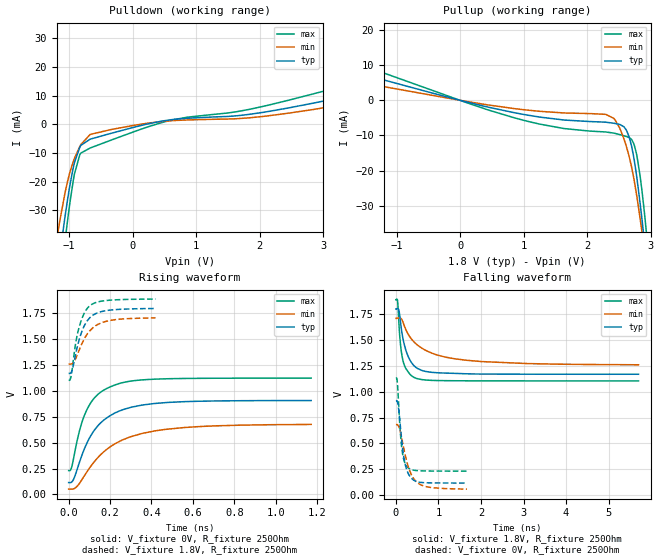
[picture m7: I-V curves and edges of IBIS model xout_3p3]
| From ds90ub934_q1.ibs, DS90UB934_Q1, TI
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|   xout_3p3 Model
[Model]   xout_3p3
Model_type   Output
Polarity   Inverting
Vmeas = 0.9
Vref = 0
Cref = 2pF
Rref = 450
|   typ   min   max
|   (nom PVT)   (fast PVT)   (slow PVT)
C_comp   3.237e-13   3.062e-13   3.274e-13
| Where nom  PVT is Nominal Process, 1.8V, 27C
|   Fast PVT is Strong Process,  1.89V, -40C
|   Slow PVT is Weak Process,   1.71V, 125C
[Voltage Range]   1.8   1.71   1.89
|Junction Temperature
[Temperature Range]   27   125   -40
[Pullup Reference]   1.8   1.71   1.89
[Pulldown Reference]   0   0   0
[Power Clamp Reference]   1.8   1.71   1.89
[GND Clamp Reference]   0   0   0
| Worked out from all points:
|   slope of the pulldown table from 0 to 0.27 V, typ, clamps not added: 188 ohm
|   slope of the pullup table from 0 to 0.27 V, typ, clamps not added: 225 ohm
|   falling waveform, V_fixture 1.8V, R_fixture 250Ohm: 20-80 % time 238ps typ, 803ps min, 133ps max; typ from 1.8 V to 1.17 V
|   rising waveform, V_fixture 0V, R_fixture 250Ohm: 20-80 % time 145ps typ, 217ps min, 101ps max; typ from 0.114 V to 0.907 V
|   rising waveform, V_fixture 1.8V, R_fixture 250Ohm: 20-80 % time 60.1ps typ, 79.4ps min, 50.6ps max; typ from 1.17 V to 1.8 V
|   falling waveform, V_fixture 0V, R_fixture 250Ohm: 20-80 % time 147ps typ, 251ps min, 97.3ps max; typ from 0.91 V to 0.116 V
[Pulldown]
|   Voltage   I(typ)   I(min)   I(max)
-3.3V     -456.4mA   -384.1mA   -520.8mA
-1.191V   -52.42mA   -39.27mA   -64.54mA
-1.063V   -31.71mA   -23.58mA   -40.14mA
-1.024V   -25.97mA   -19.69mA   -33.2mA
-938.4mV  -15.27mA   -13.06mA   -19.82mA
-826.8mV  -7.669mA   -7.408mA   -10.31mA
-670mV    -5.126mA   -3.48mA    -8.212mA
-329.7mV  -3.027mA   -1.717mA   -5.365mA
600.6mV   1.639mA    1.305mA    1.469mA
2.834V    7.407mA    5.197mA    10.63mA
4.26V     14.33mA    11.36mA    19.17mA
6.6V      27.27mA    13.11mA    34.11mA
[Pullup]
|   Voltage   I(typ)   I(min)   I(max)
-3.3V     15.02mA    10.69mA    20.67mA
856.2mV   -3.531mA   -2.361mA   -4.989mA
2.294V    -6.227mA   -3.997mA   -9.007mA
2.44V     -6.587mA   -5.567mA   -9.417mA
2.579V    -7.519mA   -10.94mA   -10.09mA
2.663V    -10.48mA   -16.05mA   -10.61mA
2.733V    -16.04mA   -21.97mA   -12.26mA
2.786V    -22.35mA   -27.65mA   -15.97mA
2.865V    -34.06mA   -37.61mA   -25.95mA
2.906V    -40.77mA   -43.25mA   -32.67mA
2.973V    -52.11mA   -52.77mA   -44.82mA
6.6V      -759.2mA   -658.7mA   -843.5mA
[Ramp]
R_load = 250
|   typ   min   max
dV/dt_r   0.477545/1.46647e-10   0.378028/2.21303e-10  0.537961/1.01561e-10
dV/dt_f   0.377772/2.3846e-10   0.26956/8.15686e-10   0.471638/1.33752e-10
[Falling Waveform]
V_fixture = 1.8V
V_fixture_min = 1.71V
V_fixture_max = 1.89V
R_fixture = 250Ohm
|   Time   V(typ)   V(min)   V(max)
0s        1.8V       1.71V      1.89V
40.63ps   1.806V     1.714V     1.871V
67.86ps   1.793V     1.714V     1.676V
102.7ps   1.689V     1.712V     1.475V
177.7ps   1.49V      1.661V     1.282V
303.3ps   1.327V     1.547V     1.184V
485.1ps   1.231V     1.46V      1.129V
969.9ps   1.185V     1.356V     1.109V
1.671ns   1.174V     1.305V     1.106V
5.704ns   1.17V      1.262V     1.105V
[Rising Waveform]
V_fixture = 0V
V_fixture_min = 0V
V_fixture_max = 0V
R_fixture = 250Ohm
|   Time   V(typ)   V(min)   V(max)
0s        114.4mV    51.01mV    229.9mV
11.63ps   115.4mV    50.33mV    245.5mV
25.05ps   151.2mV    54.71mV    360.7mV
58.81ps   349.1mV    126.1mV    661.8mV
90.21ps   504.1mV    223.9mV    826.9mV
144.9ps   671.1mV    363.6mV    972.7mV
223ps     786.3mV    488mV      1.057V
354.8ps   863.1mV    589.1mV    1.106V
485.1ps   889.2mV    631.8mV    1.118V
1.171ns   907.1mV    676mV      1.124V
[Rising Waveform]
V_fixture = 1.8V
V_fixture_min = 1.71V
V_fixture_max = 1.89V
R_fixture = 250Ohm
|   Time   V(typ)   V(min)   V(max)
0s        1.169V     1.26V      1.103V
11.63ps   1.177V     1.26V      1.141V
20ps      1.224V     1.268V     1.257V
34.22ps   1.359V     1.313V     1.464V
51.99ps   1.503V     1.4V       1.626V
74.92ps   1.627V     1.5V       1.75V
95.94ps   1.692V     1.566V     1.811V
138.8ps   1.754V     1.64V      1.859V
194.7ps   1.78V      1.679V     1.876V
419.7ps   1.797V     1.706V     1.888V
[Falling Waveform]
V_fixture = 0V
V_fixture_min = 0V
V_fixture_max = 0V
R_fixture = 250Ohm
|   Time   V(typ)   V(min)   V(max)
0s        910.3mV    681.1mV    1.127V
20ps      914.2mV    683.4mV    1.128V
34.22ps   903.5mV    681mV      1.083V
95.94ps   700.4mV    624.5mV    645.5mV
138.8ps   518.4mV    545.2mV    447.4mV
199.7ps   332.6mV    421.2mV    322.5mV
256.5ps   240.5mV    320.2mV    276.9mV
419.7ps   142.7mV    156.2mV    240.1mV
604.7ps   121.1mV    94.63mV    233.8mV
1.671ns   115.6mV    56.52mV    231mV
